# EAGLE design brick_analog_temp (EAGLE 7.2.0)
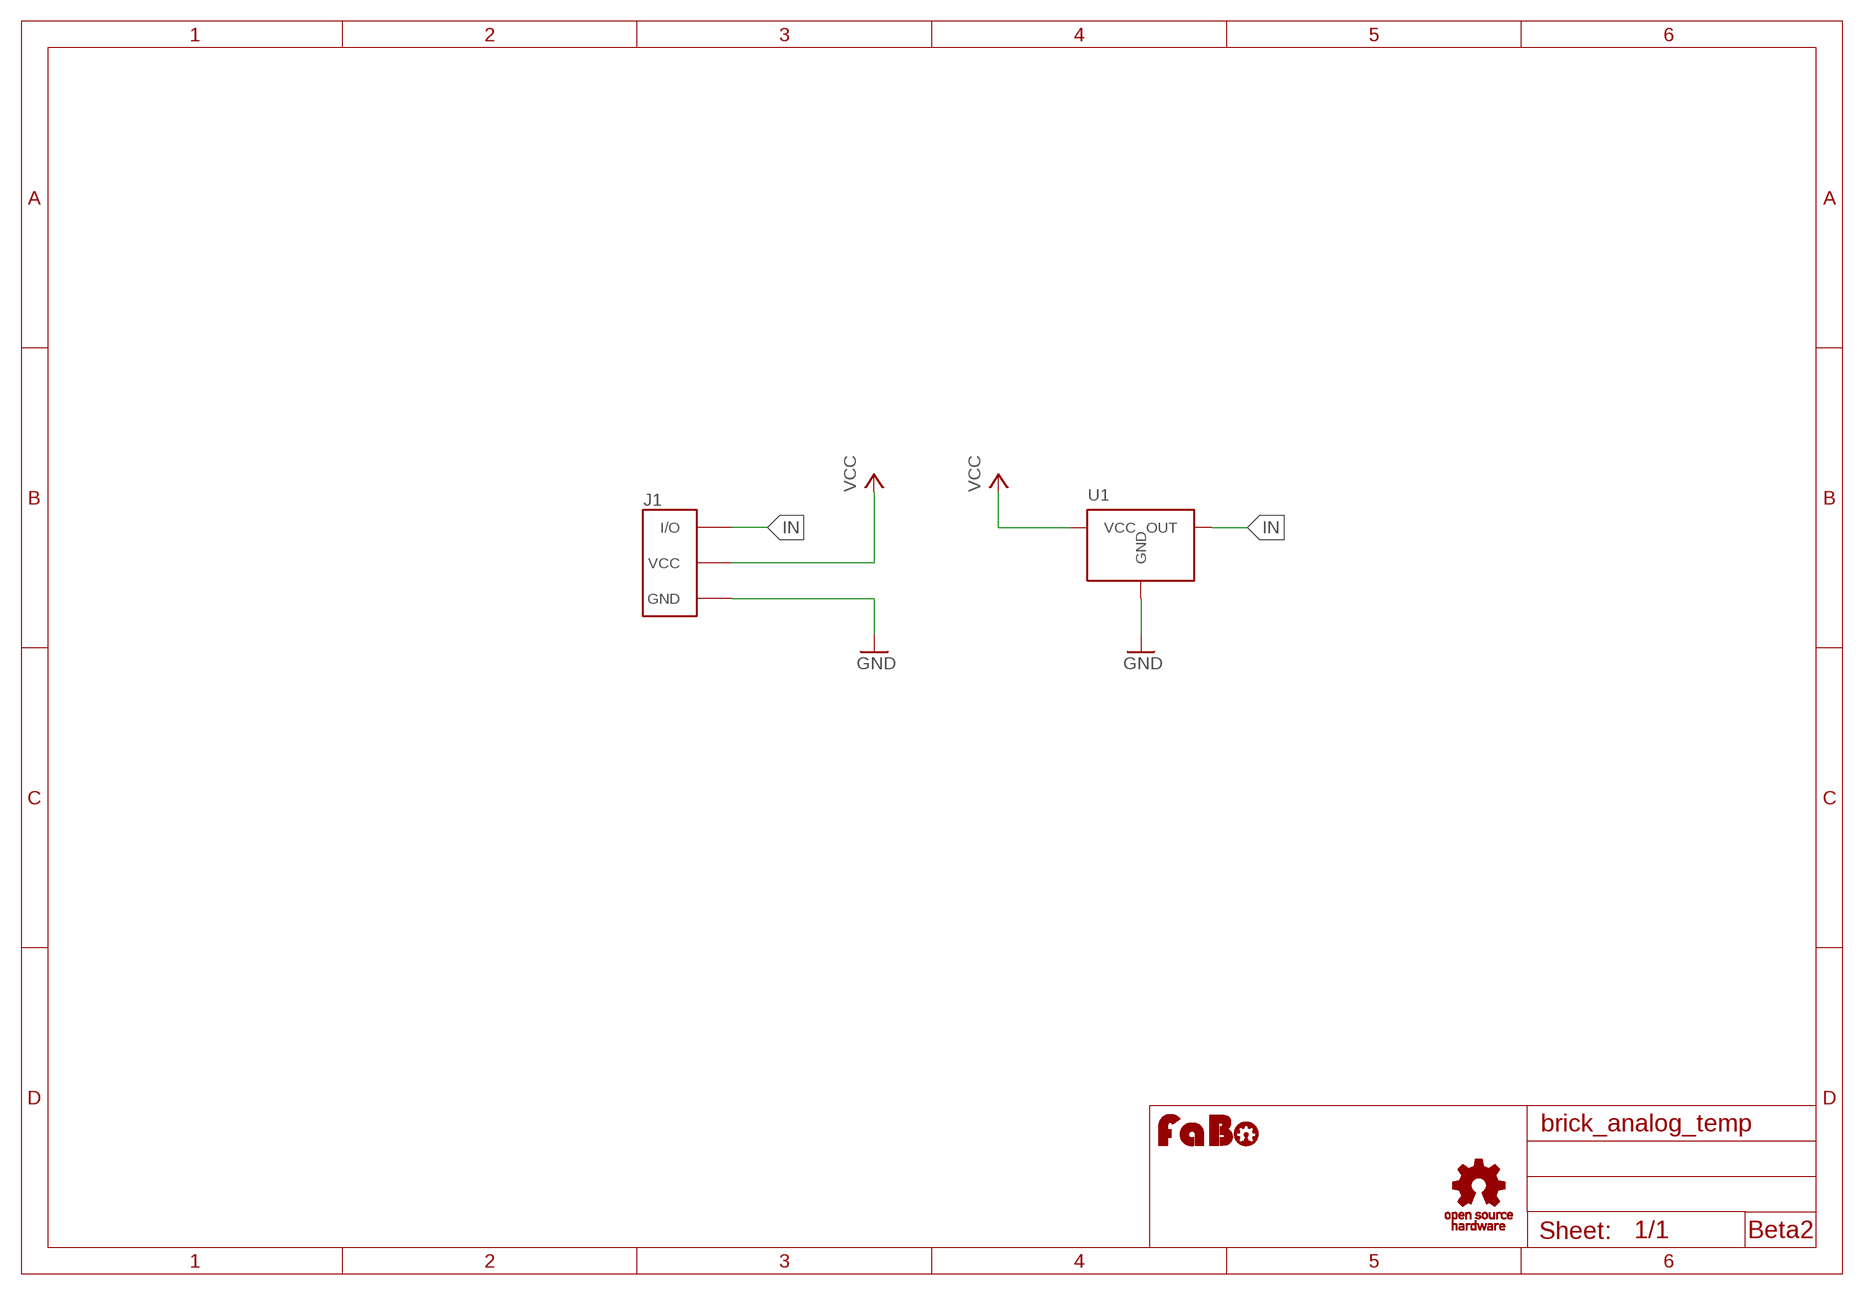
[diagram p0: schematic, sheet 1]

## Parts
J1  BRICK_3PIN  [BRICK_3PIN]
U1  SENSOR-LM60-TO92  [SENSOR-LM60-TO-92]
U$2  LOGO_OSHW_T-M  [LOGO_OSHW_T_M]
U$3  LOGO_FABO-M  [LOGO_FABO_M]

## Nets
GND: J1.GND U1.GND
IN: J1.IN/OUT(I/O) U1.OUT
VCC: J1.VCC U1.VCC

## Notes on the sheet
- Beta2

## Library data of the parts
J1 = Gclue:BRICK_3PIN: FaBo Brick 3pin
U1 = Gclue:SENSOR-LM60-: LM60 Temperature Sensor
U$2 = Gclue:LOGO_OSHW_T
U$3 = FaBo:LOGO_FABO

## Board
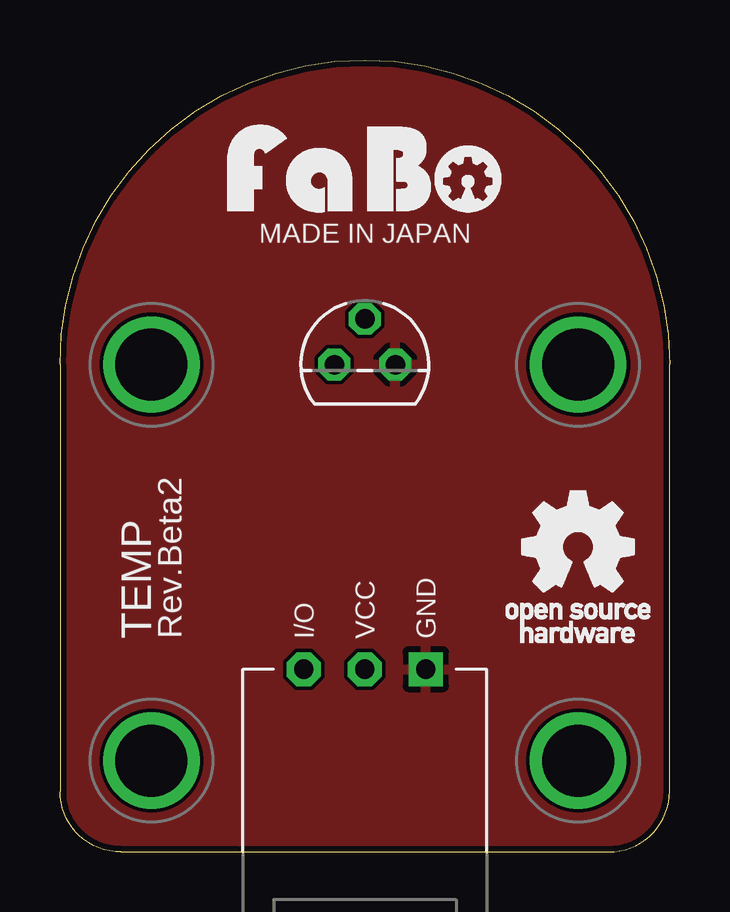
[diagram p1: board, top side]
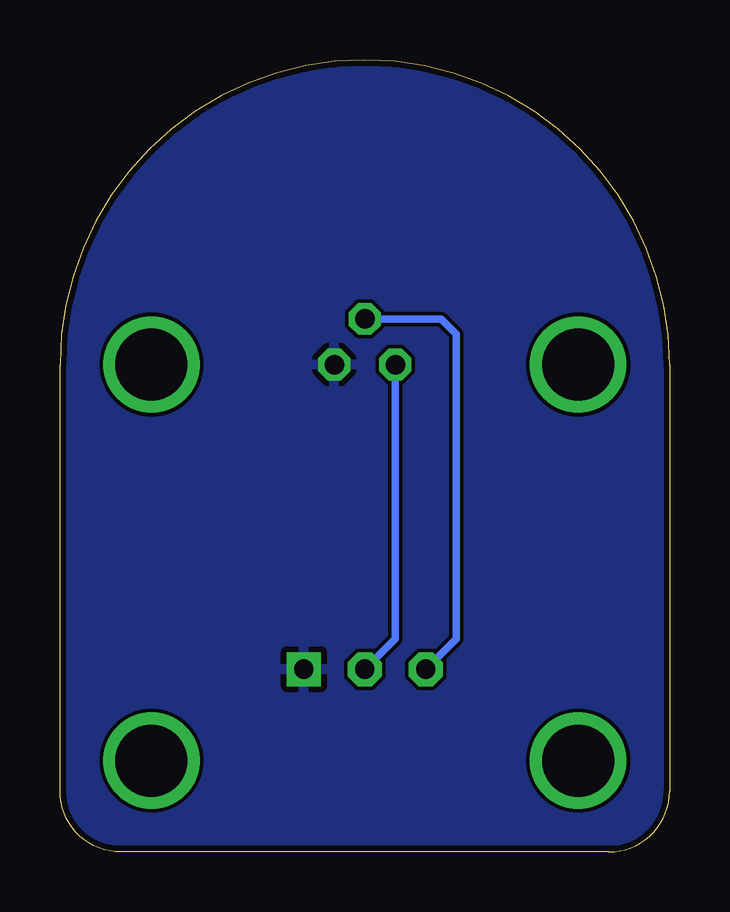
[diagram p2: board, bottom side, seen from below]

Size 25.4 x 33.02 mm. Coordinates in mm from the lower left corner, seen from the top.
Copper layers (1*16): Top 0.035mm / dielectric 1.5mm / Bottom 0.035mm
Design rules "Elecrow_2-layer_eagle_rule": minimum track width 6mil, minimum drill 12mil, track to track 6mil, track to pad 6mil, pad to pad 6mil, via to via 6mil, smd to smd 0mil, copper to edge 10mil, drill to drill 10mil, minimum pad ring 10mil, minimum via ring 6mil, stop-mask expansion 2mil, vias tented up to drill 100mil, thermal gap 10mil

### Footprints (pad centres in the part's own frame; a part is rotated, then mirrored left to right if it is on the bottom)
BRICK_3PIN = drill 0.8 pad 1.422 square: GND 2.54,-8.89 | drill 0.8 pad 1.422 octagon: IN/OUT -2.54,-8.89; VCC 0,-8.89 | drill 3 pad 3.81: P$5 -8.89,3.81; P$6 8.89,3.81; P$7 -8.89,-12.7; P$8 8.89,-12.7
SENSOR-LM60-TO-92 = drill 0.813 pad 1.27 octagon: GND 1.27,0; OUT 0,1.905; VCC -1.27,0

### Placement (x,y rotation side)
J1  12.7,16.51 0 top
U1  12.7,20.32 0 top
U$2  21.59,12.7 0 top
U$3  12.7,26.67 0 top

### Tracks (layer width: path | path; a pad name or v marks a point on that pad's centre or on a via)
GND
  pour Bottom: -1.27,-1.27 26.67,-1.27 26.67,34.29 -1.27,34.29
  pour Top: -1.27,-1.27 26.67,-1.27 26.67,34.29 -1.27,34.29
IN
  Bottom 0.305: U1.OUT 9.53,22.23 8.89,21.59 8.89,8.89 J1.IN/OUT
VCC
  Bottom 0.305: U1.VCC 11.43,8.89 J1.VCC

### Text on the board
tPlace: MADE IN JAPAN | TEMP | Rev.Beta2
